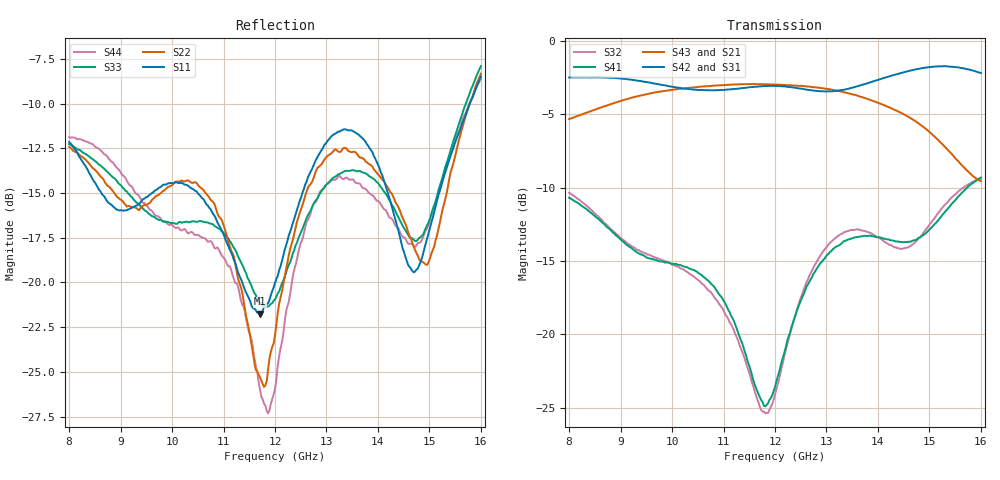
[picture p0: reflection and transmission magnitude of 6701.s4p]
# MHz S MA R 50
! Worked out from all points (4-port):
!   301 points, 8 GHz to 16 GHz, reference 50 ohm
!   strongest paths, dB at 8 GHz, 10 GHz, 12 GHz, 14 GHz, 16 GHz:
!     S42: -2.5, -3.1, -3.1, -2.7, -2.2
!     S31: -2.6, -3.2, -3.2, -2.8, -2.4
!     S43: -5.3, -3.4, -3.0, -4.2, -9.6
!     S21: -5.3, -3.5, -3.0, -4.4, -9.3
!     S41: -10.7, -15.2, -23.6, -13.4, -9.3
!     S32: -10.4, -15.2, -24.1, -13.4, -9.4
!   lowest |S11| = -21.7 dB at 11.71 GHz (marker M1), VSWR 1.18, Z = 57.1 + j5.1 ohm
!   |S11| at or under -10 dB: start of sweep to 15.78 GHz
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8000  0.2471 -173.5  0.5415 -116.6  0.7457 164.8  0.2918 -127.9
      0.5417 -116.5  0.2397 -155.3  0.3038 61.3  0.7499 -6.5
      0.7454 164.8  0.3034 61.3  0.2439 -151.5  0.5405 76.4
      0.2918 -127.9  0.7491 -6.6  0.5408 76.4  0.2549 -154.9
10613.33  0.1708 17.4  0.6891 176.9  0.6748 89.4  0.157 -174.0
          0.6891 176.8  0.181 148.5  0.1476 76.6  0.6785 -19.4
          0.6755 89.5  0.1475 76.6  0.1479 161.2  0.6983 73.8
          0.1567 -174.0  0.6784 -19.3  0.6982 73.8  0.1332 153.1
11706.67  0.08184 32.8  0.7093 146.8  0.692 60.8  0.06118 86.5
          0.7088 146.8  0.05441 -136.3  0.05687 12.0  0.6984 -22.2
          0.6925 60.8  0.05656 12.2  0.08779 -131.8  0.7111 70.8
          0.06106 86.6  0.6987 -22.1  0.7105 70.8  0.05037 -155.8
13226.67  0.2642 78.5  0.6576 104.4  0.668 19.9  0.2002 -81.8
          0.6576 104.4  0.2323 -26.2  0.2162 -128.0  0.6764 -26.9
          0.6683 19.9  0.2163 -128.0  0.2006 -2.6  0.6748 65.0
          0.2003 -81.8  0.6762 -26.9  0.6741 65.0  0.1977 -19.6
14480  0.1245 20.2  0.5617 70.0  0.7731 -15.5  0.206 -115.4
       0.5621 70.1  0.1516 -15.4  0.1962 -131.5  0.7784 -33.0
       0.7729 -15.5  0.1958 -131.4  0.144 -9.2  0.5642 59.6
       0.206 -115.5  0.7782 -33.0  0.5646 59.6  0.1341 -9.0
14960  0.1332 -66.7  0.5003 56.8  0.8032 -33.3  0.2236 -115.4
       0.5003 56.9  0.1121 -62.5  0.2309 -117.6  0.8113 -39.1
       0.8038 -33.3  0.2309 -117.6  0.1449 -63.3  0.4963 58.1
       0.2235 -115.4  0.8112 -39.1  0.4957 58.1  0.142 -54.0
16000  0.3765 -174.2  0.345 42.2  0.7632 -74.8  0.3415 -136.5
       0.3445 42.1  0.3835 -133.5  0.3389 -118.5  0.7749 -55.6
       0.7629 -74.9  0.3388 -118.5  0.4025 -119.4  0.3315 71.8
       0.3418 -136.4  0.7758 -55.6  0.3322 71.9  0.373 -120.7
